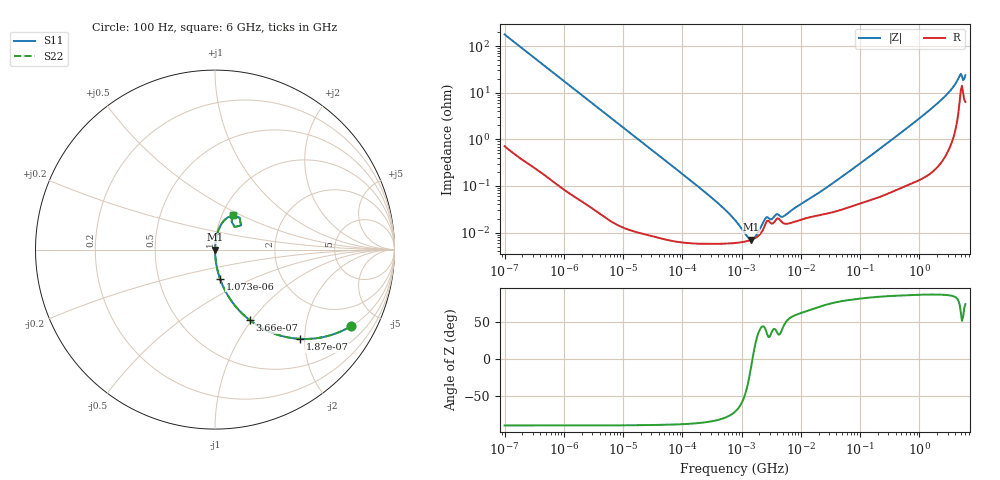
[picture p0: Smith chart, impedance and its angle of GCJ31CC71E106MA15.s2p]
!Murata Part Number: GCJ31CC71E106MA15
!These Parameters are Measured in Series Mode Connection
!Data Generated on Mar 13, 2026
!  o--ll--o
!Port1  Port2
!  o------o
!Operation Temp=25[degC], DC Bias Voltage=0[V]
!Freq. Start=100[Hz] Stop=6[GHz] 401[Steps]
# Hz S RI R 50
!Freq.(Hz) S11(Real) S11(Imag) S21(Real) S21(Imag) S12(Real) S12(Imag) S22(Real) S22(Imag)
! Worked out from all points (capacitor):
!   401 points, 100 Hz to 6 GHz, reference 50 ohm
!   read as one part in series: C = 8.95 uF near 109 Hz
!   lowest |Z| = 7.08 mohm at 1.45 MHz (marker M1)
!   series resonance near 1.526 MHz, so ESL is about 1.2 nH
!   S11 on the Smith chart (normalised r, x): 100 Hz: 1.01, -3.55; 187 Hz: 1.01, -1.90; 366 Hz: 1.00, -0.97; 1.073 kHz: 1.00, -0.33; 6 GHz: 1.13, +0.46
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100  0.7584 -0.426  0.2416 0.426  0.2416 0.426  0.7584 -0.426
187  0.4747 -0.4973  0.5253 0.4973  0.5253 0.4973  0.4747 -0.4973
366  0.1924 -0.392  0.8076 0.392  0.8076 0.392  0.1924 -0.392
573  0.0894 -0.283  0.9106 0.283  0.9106 0.283  0.0894 -0.283
1073  0.0277 -0.1618  0.9723 0.1618  0.9723 0.1618  0.0277 -0.1618
2008  0.00834 -0.0884  0.9917 0.0884  0.9917 0.0884  0.00834 -0.0884
40335  9.65e-05 -0.00447  0.9999 0.00447  0.9999 0.00447  9.65e-05 -0.00447
316350  5.73e-05 -0.000549  0.9999 0.000549  0.9999 0.000549  5.73e-05 -0.000549
774597  5.95e-05 -0.000176  0.9999 0.000176  0.9999 0.000176  5.95e-05 -0.000176
1108252  6.34e-05 -7.9e-05  0.9999 7.9e-05  0.9999 7.9e-05  6.34e-05 -7.9e-05
1449809  6.96e-05 -1.27e-05  0.9999 1.27e-05  0.9999 1.27e-05  6.96e-05 -1.27e-05
1896632  8.38e-05 5.69e-05  0.9999 -5.69e-05  0.9999 -5.69e-05  8.38e-05 5.69e-05
2594782  0.000164 0.00013  0.9998 -0.00013  0.9998 -0.00013  0.000164 0.00013
3245845  0.000155 0.000117  0.9998 -0.000117  0.9998 -0.000117  0.000155 0.000117
3882480  0.000194 0.000151  0.9998 -0.000151  0.9998 -0.000151  0.000194 0.000151
5079039  0.000159 0.000155  0.9998 -0.000155  0.9998 -0.000155  0.000159 0.000155
1.555665e7  0.000219 0.000534  0.9998 -0.000534  0.9998 -0.000534  0.000219 0.000534
3.124326e8  0.000782 0.00892  0.9992 -0.00892  0.9992 -0.00892  0.000782 0.00892
2.142435e9  0.00665 0.0624  0.9933 -0.0624  0.9933 -0.0624  0.00665 0.0624
3.352442e9  0.0191 0.1085  0.9809 -0.1085  0.9809 -0.1085  0.0191 0.1085
4.586474e9  0.072 0.1798  0.928 -0.1798  0.928 -0.1798  0.072 0.1798
6e9  0.1012 0.1932  0.8988 -0.1932  0.8988 -0.1932  0.1012 0.1932
